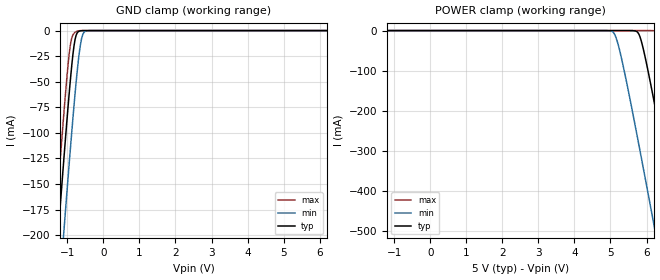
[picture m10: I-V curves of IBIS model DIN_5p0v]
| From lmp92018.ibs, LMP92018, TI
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|   Model
[Model]   DIN_5p0v
Model_type   Input
Vinl = 1.5
Vinh = 3.5
|   typ   min   max
C_comp   0.3672pF   0.3049pF   0.3707pF
[Voltage Range]   5   4.5   5.5
[Temperature Range]   27   125   -40
[Power Clamp Reference]   5   4.5   5.5
[GND Clamp Reference]   0   0   0
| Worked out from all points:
|   GND clamp passes 1 mA (typ) near -0.69 V on its own axis
[GND Clamp]
|   Voltage   I(typ)   I(min)   I(max)
-5V       -2.033A    -2.096A    -1.993A
-1.355V   -245.4mA   -317.2mA   -200mA
-1.295V   -217.1mA   -288.9mA   -171.7mA
-1.235V   -188.9mA   -260.7mA   -143.6mA
-1.085V   -120.1mA   -191.1mA   -75.79mA
-965mV    -67.9mA    -137mA     -27.99mA
-905mV    -43.97mA   -110.7mA   -11.47mA
-815mV    -14.81mA   -73.06mA   -2.667mA
-725mV    -2.117mA   -39.1mA    -519.6uA
-605mV    -108uA     -7.814mA   -19.41uA
-455mV    -1.691uA   -187.2uA   0A
9.985V    0A         0A         0A
[POWER Clamp]
|   Voltage   I(typ)   I(min)   I(max)
-5V       0A         0A         0A
5.035V    0A         -1.578mA   0A
5.275V    0A         -57.33mA   0A
5.785V    -8.459mA   -284.2mA   0A
5.935V    -55.65mA   -355.3mA   0A
6.175V    -161.1mA   -470.4mA   -150uA
6.295V    -217.1mA   -528.3mA   -1.942mA
6.475V    -302.6mA   -615.7mA   -31.45mA
6.865V    -491.2mA   -805.9mA   -204.8mA
7.375V    -740.7mA   -1.056A    -451.4mA
7.525V    -814.5mA   -1.129A    -524.8mA
9.985V    -2.025A    -2.334A    -1.739A
